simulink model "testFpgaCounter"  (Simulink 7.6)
settings: Solver=FixedStepDiscrete  StartTime=0.0  StopTime=0.1  RelTol=1e-3
PostLoadFcn:
  | set_param([gcs,'/usrp_helper'],'firmware','');
  | set_param([gcs,'/usrp_helper'],'bitstream','')
undefined symbols (not defined in the file or in its folder): array, Bit, Channels, Concatenate, D, frames, kB, kSps, Mbit, N, S, s
libraries: usrp_GPP x3, dspsnks4 x2

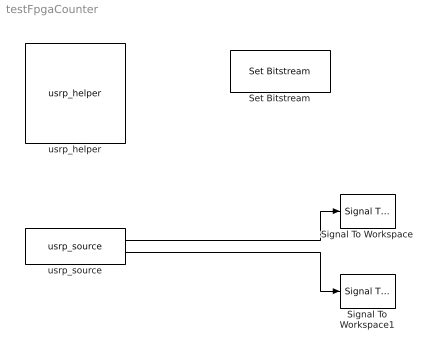
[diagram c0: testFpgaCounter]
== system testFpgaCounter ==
  Set Bitstream : usrp_GPP/Set Bitstream  SystemSampleTime=-1  bitfile=zwei.rbf
  Signal To Workspace : dspsnks4/Signal To Workspace  SystemSampleTime=-1  VariableName=Counter1  FrameMode=Concatenate frames (2-D array)
  Signal To Workspace1 : dspsnks4/Signal To Workspace  SystemSampleTime=-1  VariableName=Counter2  FrameMode=Concatenate frames (2-D array)
  usrp_helper : usrp_GPP/usrp_helper  usrp_number=0  serial_number=S/N: .  daughterboards_rx=RX A: Flex 2400 Rx, RX B: WBX NG RX,  daughterboards_tx=TX A: Flex 2400 Tx, TX B: WBX NG TX.  usb_block_size=0  usb_nblocks=0  firmware=C:\Users\nagel\Documents\sff_sdr\Simulink-USRP\simulink-usrp_2.1.0\firmware\rev4\std.ihx  bitstream=C:\Users\nagel\Documents\sff_sdr\Simulink-USRP\simulink-usrp_2.1.0\firmware\rev4\fpgaCounter.rbf  sample_time_factor=1
  usrp_source : usrp_GPP/usrp_source  usrp_number=0  serial_number=S/N: .  decimation=256  sample_width=16 Bit  sampling_rate_and_bandwidth=1 Channels: 250 kSps, 976.563 kB/s, 7.62939 Mbit/s.  vector_length=1024  sideA_subdev1_tab_=0  sideA_subdev1_subdevice=Flex 2400 Rx  sideA_subdev1_datatype=INT16  sideA_subdev1_frequency_range=Min: 2.3 GHz, Max: 2.9 GHz.  sideA_subdev1_frequency_port=off  sideA_subdev1_frequency=2.4e9  sideA_subdev1_gain_range=Min: 0 dB, Max: 90 dB, Step Size: 0.05 dB.  sideA_subdev1_gain=0  sideA_subdev1_antenna=Not applicable  sideA_subdev2_tab_=0  sideA_subdev2_subdevice=Not available.  sideA_subdev2_datatype=Disabled  sideA_subdev2_frequency_range=Unknown.  sideA_subdev2_frequency_port=off  sideA_subdev2_frequency=0  sideA_subdev2_gain_range=Unknown.  sideA_subdev2_gain=0  sideB_subdev1_tab_=0  sideB_subdev1_subdevice=WBX NG RX  sideB_subdev1_datatype=Disabled  sideB_subdev1_frequency_range=Min: 68.75 MHz, Max: 2.2 GHz.  sideB_subdev1_frequency_port=off  sideB_subdev1_frequency=0  sideB_subdev1_gain_range=Min: 0 dB, Max: 50.5 dB, Step Size: 0.05 dB.  sideB_subdev1_gain=0  sideB_subdev1_antenna=Not applicable  sideB_subdev2_subdevice=Not available.  sideB_subdev2_datatype=Disabled  sideB_subdev2_frequency_range=Unknown.  sideB_subdev2_frequency_port=off  sideB_subdev2_frequency=0  sideB_subdev2_gain_range=Unknown.  sideB_subdev2_gain=0
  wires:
  usrp_source/1 -> Signal To Workspace/1
  usrp_source/2 -> Signal To Workspace1/1
